(* Logix 5000 DataType export ToloOutput; software revision 20.01 *)

TYPE ToloOutput :
STRUCT
   Control : SINT;
   Move_Select : SINT;
   Target_0_Position : REAL;
   Target_0_Velocity : REAL;
   Target_0_Acceleration : REAL;
   Target_0_Deceleration : REAL;
   Target_0_Force : REAL;
   Motion_Type : SINT;
   Digital_Output : DINT;
END_STRUCT
END_TYPE
